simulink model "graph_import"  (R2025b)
settings: Solver=VariableStepAuto  StartTime=0.0  StopTime=10  RelTol=1e-3
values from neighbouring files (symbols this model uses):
  S = sum(round(C0))    [NormalizeCoef.m]
undefined symbols (not defined in the file or in its folder): AIE, code, Connector, Evaluation, FMC, ML, netlist, Platform, VEK280, Versal, vsvh1760, with, xcve2802
libraries: vmcUtilities x1, dspsrcs4 x1, aieUtilities x1

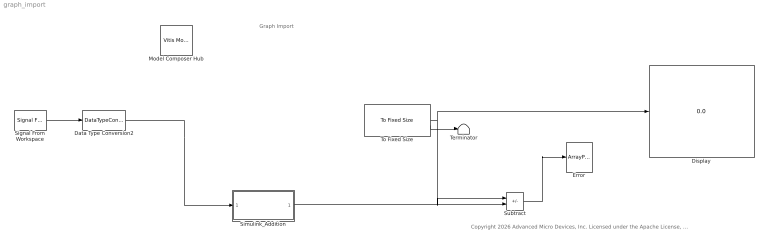
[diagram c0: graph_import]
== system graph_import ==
  note: Graph Import
  note: Copyright 2026 Advanced Micro Devices, Inc. Licensed under the Apache License, Version 2.0 (the "License"); you may not use this file except in compliance with the License. You may obtain a copy of the License at http://www.apache.org/licenses/LICENSE-2.0 Unless required by applicable law or agreed to in writing, software distributed under the License is distributed on an "AS IS" BASIS, WITHOUT WARRANTIES OR CONDITIONS OF ANY KIND, either express or implied. See the License for the specific language governing permissions and limitations under the License.
  Data Type Conversion2 : DataTypeConversion  OutDataTypeStr=int16
  Display : Display
  Error : ArrayPlot  WindowPosition=[913.000000,318.000000,845.000000,423.000000,]  ScopeFrameLocation=window  PlotType=Line  ShowLegend=on
  Model Composer Hub : vmcUtilities/Vitis Model Composer Hub  Tag=genX  CodeGeneration=off  SubsystemName=DUT  StartColumn=1  NumberOfColumns=1  TargetDirectory=./code  exportDesign=off  analyzeDesign=off  validateDesignOnHw=off  ExportType=AI Engines  IpVendor=xilinx.com  IpLibrary=hls  IpVersion=1.0  IpHWLanguage=Verilog  AieCompilerOptions={}  AieSimulatorOptions={}  CreateTestbench=on  TestbenchStackSize=10  RunRtlSim=off  RunCSim=off  RunAieSim=on  AieSimTimeout=50000  RunAieSimProfiling=off  LaunchVitisAnalyzer=off  PlotOutput=off  RunX86Sim=off  X86SimTimeout=10  GenHwImage=off  GenLibadfXo=off  GenHwValidationCode=off  PlatformType=Specify Platform  Platform=/opt/amd/2025.2/Vitis/base_platforms/xilinx_vek280_base_202520_1/xilinx_vek280_base_202520_1.xpfm  HwSystemType=Baremetal  HwValidationTarget=hw  ProjDevice=Versal VEK280 Evaluation Platform with FMC Connector (xcve2802-vsvh1760-2MP-e-S)  ProjDevicePart=xcve2802-vsvh1760-2MP-e-S  AIEType=AIE-ML  SamplePeriod=-1  ClockFrequency=200  DataPathParallelism=1  xilinxfamily=versalaiedge  part=xcve2802  speed=-2MP-e-S  package=vsvh1760  directory=./netlist  testbench=off  incr_netlist=off  synthesis_tool=Vivado  clock_wrapper=Clock Enables  dbl_ovrd=According to Block Masks  dcm_input_clock_period=10  sysclk_period=10  simulink_period=1  eval_field=0  IPInfoJsonString="{\"AIESubsystem\":{\"SubsystemName\":\"DUT\",\"TargetDirectory\":\"./code\",\"SubsystemDir\":\"./code/ip/DUT\"}}"  LogFileName=/proj/xsjhdstaff4/abehbood/vmc_examples/gitent2/Examples/AIENGINE/Importing_AIE_blocks/AIE_Graph/code/model_composer.log  NThreads=4
  Signal From Workspace : dspsrcs4/Signal From Workspace  X=1:16  Ts=1  nsamps=16  OutputAfterFinalValue=Setting to zero  ignoreOrWarnInputAndFrameLengths=off  OutputFrames=off
  Simulink_Addition : Subsystem
  Subtract : Sum  Inputs=+-
  Terminator : Terminator
  To Fixed Size : aieUtilities/To Fixed Size  Mode=Produce a valid output signal  OutputSize=Inherit: Same as input  CopyMethod=Buffer samples to form output  HasStatusOutput=on
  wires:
  To Fixed Size/1 -> Subtract/1, Display/1
  Signal From Workspace/1 -> Data Type Conversion2/1
  Simulink_Addition/1(Out1) -> Subtract/2
  Subtract/1 -> Error/1
  Data Type Conversion2/1 -> Simulink_Addition/1(In1)
  To Fixed Size/2 -> Terminator/1
  ? -> To Fixed Size/1

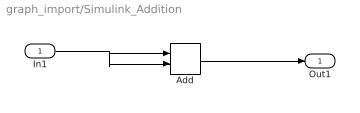
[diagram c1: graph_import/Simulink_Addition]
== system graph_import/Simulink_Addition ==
  In1 : Inport
  Add : Sum
  Out1 : Outport
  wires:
  In1/1 -> Add/2, Add/1
  Add/1 -> Out1/1
